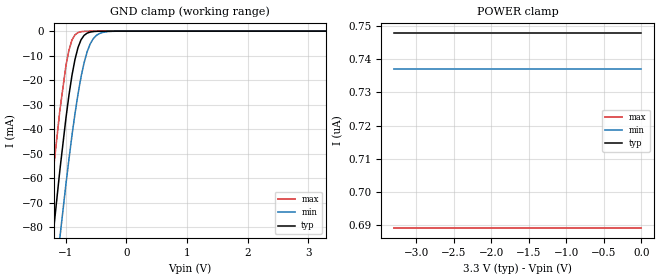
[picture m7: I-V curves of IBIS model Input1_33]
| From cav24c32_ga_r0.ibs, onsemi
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|//////////////////////////////////////////////////////////////////////////////
|//////////////////////////////////////////////////////////////////////////////
[Model]  Input1_33
Model_type Input
Vinh = 2.31
Vinl = 0.99
|  variable   typ   min   max
C_comp   6pF   6pF   6pF
|//////////////////////////////////////////////////////////////////////////////
[Temperature Range]   25   125   -40
|//////////////////////////////////////////////////////////////////////////////
[Voltage Range]   3.30V   3.00V   3.60V
|//////////////////////////////////////////////////////////////////////////////
[POWER Clamp Reference] 3.30V   3.00V   3.60V
|//////////////////////////////////////////////////////////////////////////////
[GND Clamp Reference]   0V   0V   0V
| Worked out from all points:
|   GND clamp passes 1 mA (typ) near -0.66 V on its own axis
|//////////////////////////////////////////////////////////////////////////////
[GND Clamp]
|   Voltage   I(typ)   I(min)   I(max)
-3.3V     -668mA     -676mA     -661mA
-1.3V     -105mA     -132mA     -80.1mA
-1.2V     -80.2mA    -108mA     -55.1mA
-1.1V     -56.7mA    -84.3mA    -32.3mA
-1V       -35.5mA    -62.4mA    -14.1mA
-950mV    -26.1mA    -52.2mA    -7.69mA
-900mV    -18mA      -42.5mA    -3.61mA
-800mV    -6.64mA    -25.6mA    -575uA
-700mV    -1.72mA    -12.9mA    -90.4uA
-600mV    -376uA     -5.25mA    -24.7uA
-400mV    -23.3uA    -565uA     -10.1uA
3.3V      748nA      737nA      689nA
|//////////////////////////////////////////////////////////////////////////////
[POWER Clamp]
|   Voltage   I(typ)   I(min)   I(max)
-3.3V     748nA      737nA      689nA
-3.2V     748nA      737nA      689nA
-3.1V     748nA      737nA      689nA
0V        748nA      737nA      689nA
